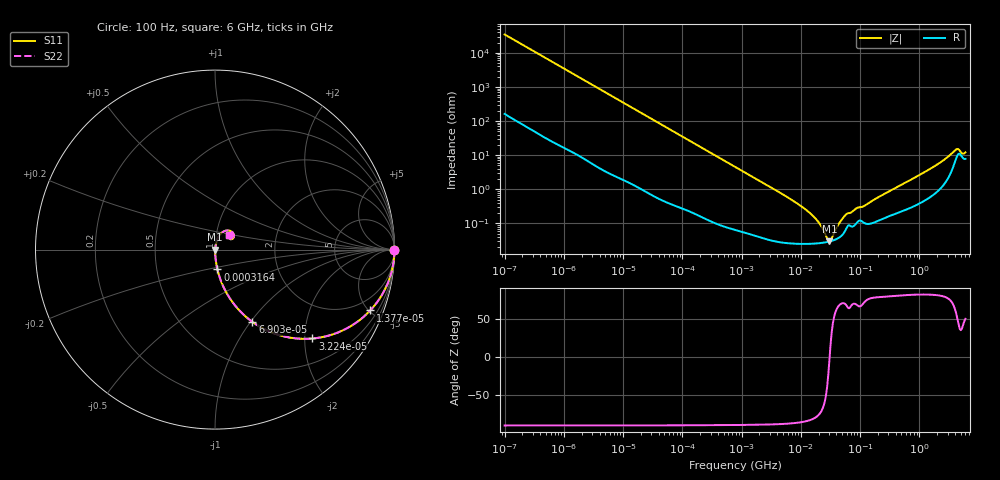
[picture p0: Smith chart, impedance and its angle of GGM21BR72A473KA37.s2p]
!Murata Part Number: GGM21BR72A473KA37
!These Parameters are Measured in Series Mode Connection
!Data Generated on Mar 13, 2026
!  o--ll--o
!Port1  Port2
!  o------o
!Operation Temp=25[degC], DC Bias Voltage=0[V]
!Freq. Start=100[Hz] Stop=6[GHz] 401[Steps]
# Hz S RI R 50
!Freq.(Hz) S11(Real) S11(Imag) S21(Real) S21(Imag) S12(Real) S12(Imag) S22(Real) S22(Imag)
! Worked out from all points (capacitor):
!   401 points, 100 Hz to 6 GHz, reference 50 ohm
!   read as one part in series: C = 46 nF near 109 Hz
!   lowest |Z| = 29.5 mohm at 30.45 MHz (marker M1)
!   series resonance near 30.65 MHz, so ESL is about 590 pH
!   S11 on the Smith chart (normalised r, x): 100 Hz: open; 13.77 kHz: 1.03, -5.09; 32.24 kHz: 1.01, -2.18; 69.03 kHz: 1.01, -1.02; 316.4 kHz: 1.00, -0.22; 6 GHz: 1.16, +0.18
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100  1 -0.00289  2.2e-05 0.00289  2.2e-05 0.00289  1 -0.00289
2008  0.9964 -0.0574  0.00359 0.0574  0.00359 0.0574  0.9964 -0.0574
5625  0.974 -0.1566  0.026 0.1566  0.026 0.1566  0.974 -0.1566
13772  0.8648 -0.3391  0.1352 0.3391  0.1352 0.3391  0.8648 -0.3391
32244  0.5429 -0.4952  0.4571 0.4952  0.4571 0.4952  0.5429 -0.4952
40335  0.4325 -0.4924  0.5675 0.4924  0.5675 0.4924  0.4325 -0.4924
69028  0.2084 -0.4027  0.7916 0.4027  0.7916 0.4027  0.2084 -0.4027
129199  0.0714 -0.2534  0.9286 0.2534  0.9286 0.2534  0.0714 -0.2534
316350  0.0135 -0.1106  0.9865 0.1106  0.9865 0.1106  0.0135 -0.1106
774597  0.00275 -0.0459  0.9972 0.0459  0.9972 0.0459  0.00275 -0.0459
6644369  0.000285 -0.00518  0.9997 0.00518  0.9997 0.00518  0.000285 -0.00518
1.555665e7  0.000256 -0.00173  0.9997 0.00173  0.9997 0.00173  0.000256 -0.00173
2.035112e7  0.000263 -0.000998  0.9997 0.000998  0.9997 0.000998  0.000263 -0.000998
2.784235e7  0.000284 -0.000229  0.9997 0.000229  0.9997 0.000229  0.000284 -0.000229
3.045065e7  0.000295 -1.55e-05  0.9997 1.55e-05  0.9997 1.55e-05  0.000295 -1.55e-05
3.330331e7  0.000307 0.000199  0.9997 -0.000199  0.9997 -0.000199  0.000307 0.000199
4.556224e7  0.000396 0.001  0.9996 -0.001  0.9996 -0.001  0.000396 0.001
5.699437e7  0.000642 0.00166  0.9994 -0.00166  0.9994 -0.00166  0.000642 0.00166
3.124326e8  0.00171 0.0086  0.9983 -0.0086  0.9983 -0.0086  0.00171 0.0086
1.712697e9  0.00866 0.0436  0.9913 -0.0436  0.9913 -0.0436  0.00866 0.0436
4.009986e9  0.0728 0.1072  0.9272 -0.1072  0.9272 -0.1072  0.0728 0.1072
6e9  0.0787 0.0786  0.9213 -0.0786  0.9213 -0.0786  0.0787 0.0786
